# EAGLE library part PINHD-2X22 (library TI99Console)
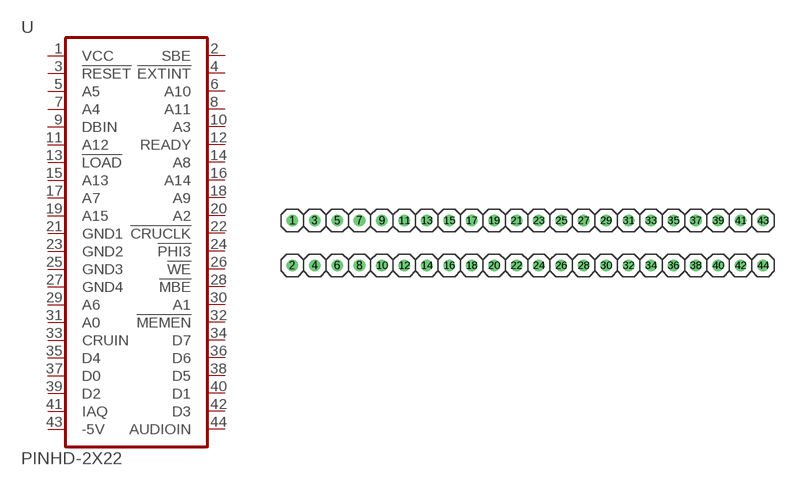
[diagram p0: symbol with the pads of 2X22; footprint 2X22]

Designator prefix -

## PINHD-2X22  [2X22]
1  VCC  pwr
2  SBE  out
3  !RESET  out
4  !EXTINT  in
5  A5  out
6  A10  out
7  A4  out
8  A11  out
9  DBIN  out
10  A3  out
11  A12  out
12  READY  out
13  !LOAD  out
14  A8  out
15  A13  out
16  A14  out
17  A7  out
18  A9  out
19  A15  out
20  A2  out
21  GND1  pwr
22  !CRUCLK  out
23  GND2  pwr
24  !PHI3  out
25  GND3  pwr
26  !WE  out
27  GND4  pwr
28  !MBE  out
29  A6  out
30  A1  out
31  A0  out
32  !MEMEN  out
33  CRUIN  in
34  D7
35  D4
36  D6
37  D0
38  D5
39  D2
40  D1
41  IAQ  out
42  D3
43  -5V  pwr
44  AUDIOIN  in

## Footprint 2X22 (pad centres in mm)
drill 0.8: 1 -26.67,0; 2 -26.67,-5.08; 3 -24.13,0; 4 -24.13,-5.08; 5 -21.59,0; 6 -21.59,-5.08; 7 -19.05,0; 8 -19.05,-5.08; 9 -16.51,0; 10 -16.51,-5.08; 11 -13.97,0; 12 -13.97,-5.08; 13 -11.43,0; 14 -11.43,-5.08; 15 -8.89,0; 16 -8.89,-5.08; 17 -6.35,0; 18 -6.35,-5.08; 19 -3.81,0; 20 -3.81,-5.08; 21 -1.27,0; 22 -1.27,-5.08; 23 1.27,0; 24 1.27,-5.08; 25 3.81,0; 26 3.81,-5.08; 27 6.35,0; 28 6.35,-5.08; 29 8.89,0; 30 8.89,-5.08; 31 11.43,0; 32 11.43,-5.08; 33 13.97,0; 34 13.97,-5.08; 35 16.51,0; 36 16.51,-5.08; 37 19.05,0; 38 19.05,-5.08; 39 21.59,0; 40 21.59,-5.08; 41 24.13,0; 42 24.13,-5.08; 43 26.67,0; 44 26.67,-5.08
